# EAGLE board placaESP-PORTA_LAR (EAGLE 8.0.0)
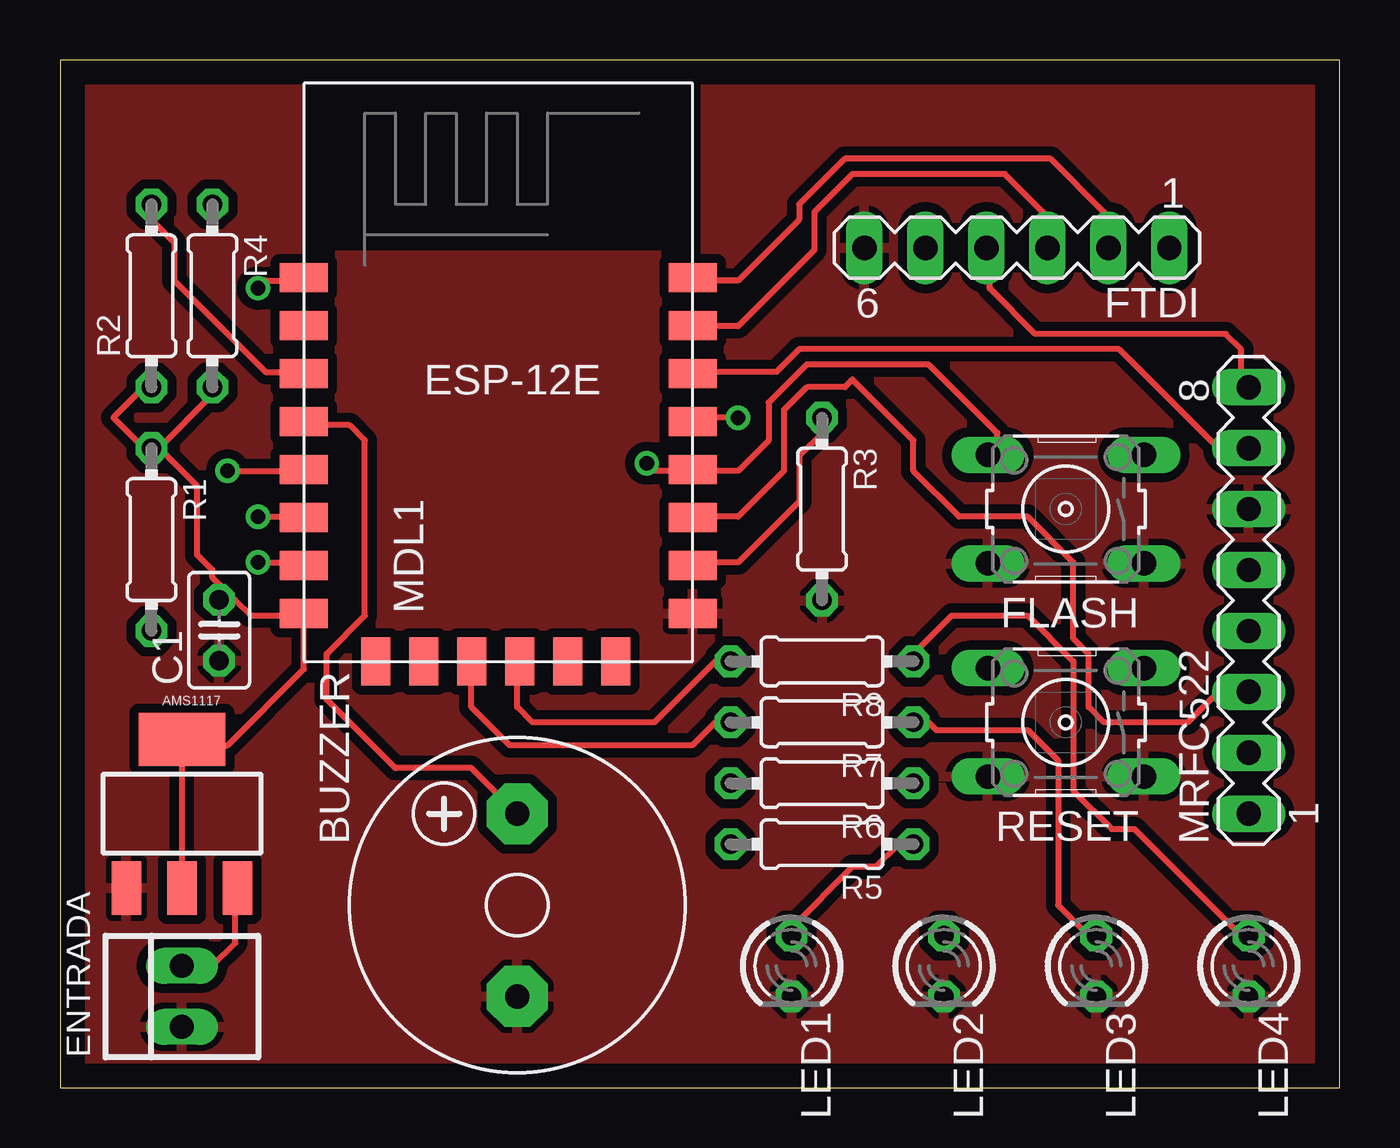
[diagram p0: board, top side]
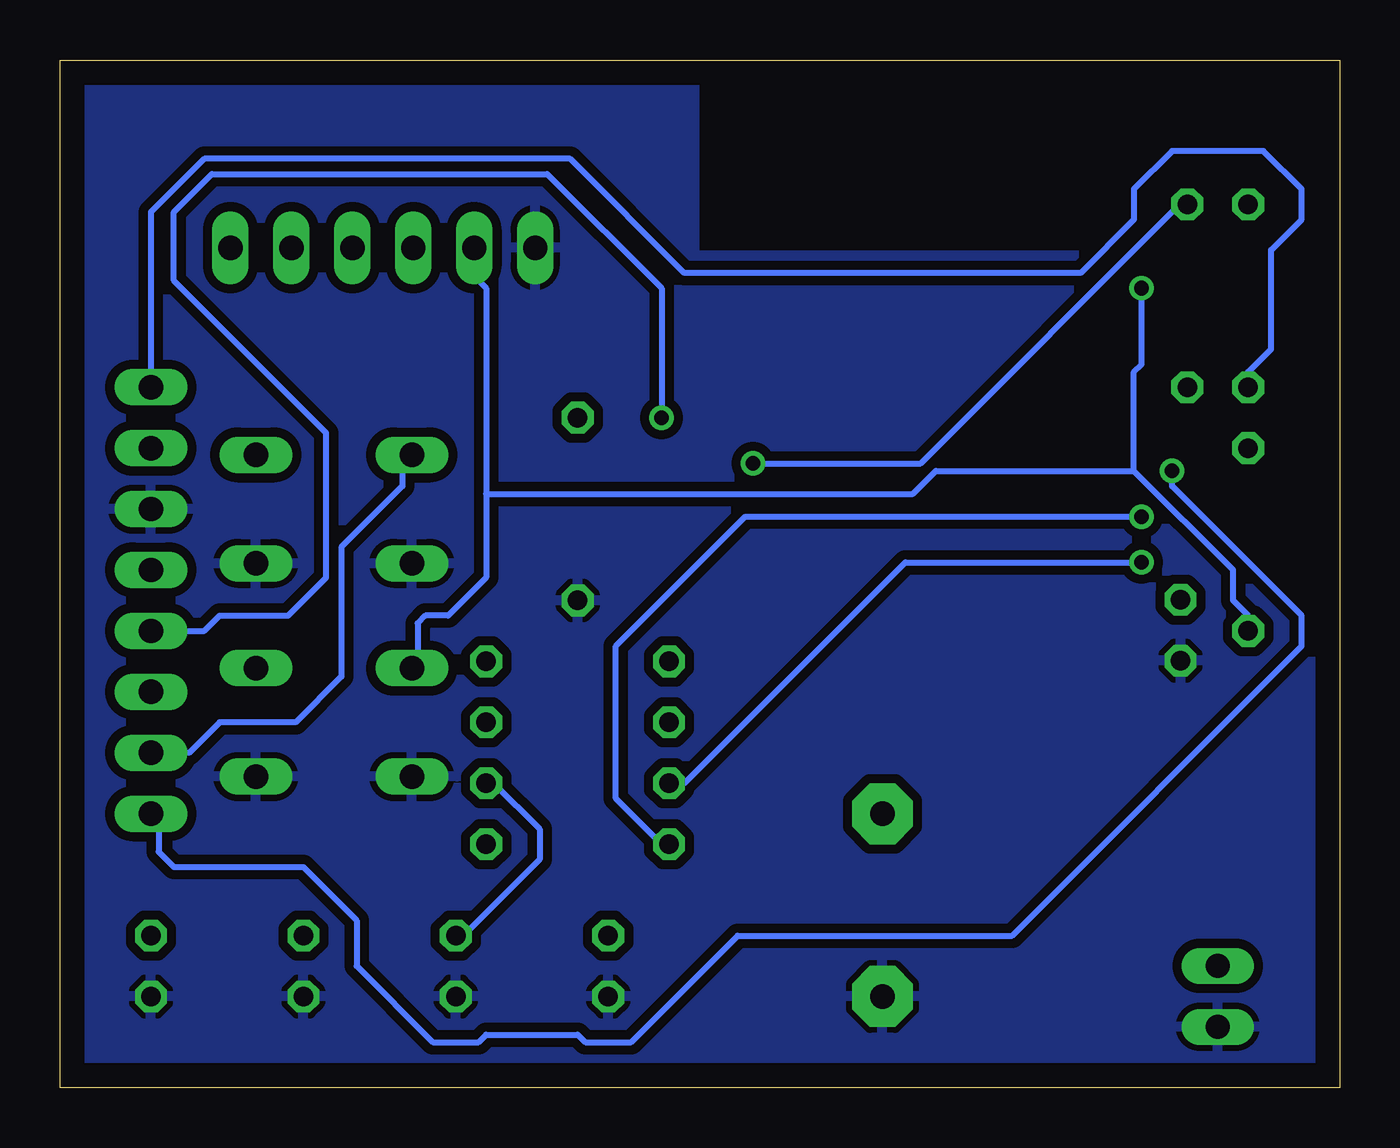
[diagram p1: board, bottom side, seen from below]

Size 53.32 x 42.85 mm. Coordinates in mm from the lower left corner, seen from the top.
Outline: 0,0 53.32,0 53.32,42.85 0,42.85 0,0
Copper layers (1*16): Top 0.035mm / dielectric 1.5mm / Bottom 0.035mm
Design rules "default *": minimum track width 10mil, minimum drill 24mil, track to track 15mil, track to pad 15mil, pad to pad 15mil, via to via 15mil, smd to smd 8mil, copper to edge 40mil, drill to drill 8mil, minimum pad ring 10mil, minimum via ring 8mil, stop-mask expansion 4mil, vias tented up to drill 0mil, thermal gap 10mil

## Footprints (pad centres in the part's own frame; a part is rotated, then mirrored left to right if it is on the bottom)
AMS1117 = smd 1.219 x 2.235: GND -2.311,-3.099; VIN 2.311,-3.099; VOUT 0,-3.099 | smd 3.6 x 2.2: HEATSINK 0,3.099
F/CM12P = drill 1.016 pad 2.54 octagon: + 3.81,0; - -3.81,0
C025-025X050 = drill 0.813 octagon: 1 -1.27,0; 2 1.27,0
22-23-2021 = drill 1 long: 1 -1.27,0; 2 1.27,0
B3F-10XX = drill 1.016 long: 1 -3.251,2.261; 2 3.251,2.261; 3 -3.251,-2.261; 4 3.251,-2.261
MA06-1 = drill 1.016 long: 1 -6.35,0; 2 -3.81,0; 3 -1.27,0; 4 1.27,0; 5 3.81,0; 6 6.35,0
LED3MM = drill 0.813 octagon: A -1.27,0; K 1.27,0
ESP8266-ESP12E = smd 2 x 1.2: 1 -7.62,5.84; 2 -7.62,3.84; 3 -7.62,1.84; 4 -7.62,-0.16; 5 -7.62,-2.16; 6 -7.62,-4.16; 7 -7.62,-6.16; 8 -7.62,-8.16; 9 8.58,-8.16; 10 8.58,-6.16; 11 8.58,-4.16; 12 8.58,-2.16; 13 8.58,-0.16; 14 8.58,1.84; 15 8.58,3.84; 16 8.58,5.84 | smd 1.2 x 2: 17 -4.62,-10.16; 18 -2.62,-10.16; 19 -0.62,-10.16; 20 1.38,-10.16; 21 3.38,-10.16; 22 5.38,-10.16
MA08-1 = drill 1.016 long: 1 -8.89,0; 2 -6.35,0; 3 -3.81,0; 4 -1.27,0; 5 1.27,0; 6 3.81,0; 7 6.35,0; 8 8.89,0
0204/7 = drill 0.813 octagon: 1 -3.81,0; 2 3.81,0

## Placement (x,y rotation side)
AMS1117  [AMS1117]  5.08,11.43 0 top
BUZZER  F/CM12P  [F/CM12P]  19.05,7.62 90 top
C1  100n  [C025-025X050]  6.63,19.08 90 top
ENTRADA  22-23-2021  [22-23-2021]  5.08,3.81 90 top
FLASH  [B3F-10XX]  41.91,24.13 180 top
FTDI  [MA06-1]  39.87,35.02 180 top
LED1  [LED3MM]  30.48,5.08 270 top
LED2  [LED3MM]  36.83,5.08 270 top
LED3  [LED3MM]  43.18,5.08 270 top
LED4  [LED3MM]  49.53,5.08 270 top
MDL1  [ESP8266-ESP12E]  17.78,27.94 0 top
MRFC522  [MA08-1]  49.53,20.32 90 top
R1  10k  [0204/7]  3.81,22.86 270 top
R2  10k  [0204/7]  3.81,33.02 90 top
R3  10k  [0204/7]  31.75,24.13 270 top
R4  10k  [0204/7]  6.35,33.02 270 top
R5  220R  [0204/7]  31.75,10.16 180 top
R6  220R  [0204/7]  31.75,12.7 180 top
R7  220R  [0204/7]  31.75,15.24 180 top
R8  220R  [0204/7]  31.75,17.78 180 top
RESET  [B3F-10XX]  41.91,15.24 180 top

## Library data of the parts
AMS1117 = kaibader
BUZZER = buzzer; OC_FARNELL: unknown; OC_NEWARK: unknown
C1 = rcl
ENTRADA = con-molex; MF: MOLEX; MPN: 22-23-2021; OC_FARNELL: 1462926; OC_NEWARK: 25C3832
FLASH RESET = switch-omron; MPN: B3F-1000; OC_FARNELL: 176432; OC_NEWARK: 36M3542
FTDI MRFC522 = con-lstb; OC_FARNELL: unknown; OC_NEWARK: unknown
LED1-LED4 = led
MDL1 = ESP8266-ESP12E
R1-R8 = resistor

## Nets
BUZZ: BUZZER.+ MDL1.4
CTS: FTDI.5 MDL1.1 R1.2 RESET.4
DTR: FTDI.1
GND: AMS1117.GND BUZZER.- C1.1 ENTRADA.1 FLASH.1 FLASH.2 FTDI.6 LED1.K LED2.K LED3.K LED4.K MDL1.9 MRFC522.6 R3.2 RESET.1 RESET.2
IN+: AMS1117.VIN ENTRADA.2
IRQ: MRFC522.5
LED1: MDL1.6 R5.2
LED2: MDL1.7 R6.2
LED3: MDL1.19 R7.2
LED4: MDL1.20 R8.2
MISO: MDL1.13 MRFC522.4
MOSI: MDL1.11 MRFC522.3
N$1: MDL1.10 R3.1
N$3: MDL1.3 R2.2
N$5: LED1.A R5.1
N$6: LED2.A R6.1
N$7: LED3.A R7.1
N$8: LED4.A R8.1
RST: MDL1.14 MRFC522.7
RXI: FTDI.2 MDL1.16
SCK: FLASH.4 MDL1.12 MRFC522.2 R4.1
SDA: MDL1.5 MRFC522.1
TXO: FTDI.3 MDL1.15
VCC: AMS1117.HEATSINK AMS1117.VOUT C1.2 FTDI.4 MDL1.8 MRFC522.8 R1.1 R2.1 R4.2

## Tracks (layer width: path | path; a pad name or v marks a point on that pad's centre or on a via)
BUZZ
  Top 0.254: BUZZER.+ 17.14,13.34 13.97,13.34 11.11,16.19 11.11,18.1 12.7,19.68 12.7,26.99 12.06,27.62 10.16,27.62 MDL1.4
CTS  (via drill 0.61)
  Top 0.254: v8.26,33.34 8.57,33.66 10.16,33.66 MDL1.1
  Bottom 0.254: v8.26,33.34 8.26,30.16 8.57,29.84 8.57,25.72 | 8.57,25.72 4.45,21.59 4.45,20.32 3.81,19.68 R1.2 | 35.56,24.77 35.56,33.34 35.88,33.66 35.88,34.92 FTDI.5 | 35.56,24.77 35.56,21.27 37.15,19.68 38.1,19.68 38.42,19.37 38.42,17.78 RESET.4 | 8.57,25.72 16.83,25.72 17.78,24.77 35.56,24.77
GND
  pour Bottom: 0,0 53.35,0 53.35,42.79 0,42.79
  pour Top: 0,0 53.3,0 53.3,42.84 0,42.84
IN+
  Top 0.254: ENTRADA.2 6.35,5.08 7.3,6.03 7.3,8.26 AMS1117.VIN
LED1  (via drill 0.61)
  Top 0.254: v8.26,23.81 10.16,23.81 MDL1.6
  Bottom 0.254: v8.26,23.81 24.77,23.81 30.16,18.41 30.16,12.06 28.26,10.16 R5.2
LED2  (via drill 0.61)
  Top 0.254: v8.26,21.91 10.16,21.91 MDL1.7
  Bottom 0.254: v8.26,21.91 18.1,21.91 27.3,12.7 R6.2
LED3
  Top 0.254: R7.2 27.3,15.24 26.35,14.29 18.73,14.29 17.14,15.88 17.14,17.78 MDL1.19
LED4
  Top 0.254: R8.2 27.3,17.78 24.77,15.24 19.68,15.24 19.05,15.88 19.05,17.78 MDL1.20
MISO  (via drill 0.61)
  Top 0.254: v28.26,27.94 26.67,27.94 MDL1.13
  Bottom 0.254: v28.26,27.94 28.26,33.34 33.02,38.1 46.99,38.1 48.58,36.51 48.58,33.66 42.23,27.3 42.23,21.27 43.81,19.68 46.67,19.68 47.31,19.05 MRFC522.4
MOSI
  Top 0.254: MRFC522.3 48.26,16.51 46.99,15.24 43.5,15.24 42.86,15.88 42.86,18.1 42.23,18.73 42.23,21.91 40.32,23.81 37.47,23.81 35.56,25.72 35.56,26.99 33.02,29.53 32.7,29.21 31.11,29.21 30.16,28.26 30.16,25.72 28.26,23.81 26.67,23.81 MDL1.11
N$1
  Top 0.254: R3.1 31.75,27.3 30.8,26.35 30.8,24.45 28.26,21.91 26.67,21.91 MDL1.10
N$3
  Top 0.254: R2.2 3.81,36.2 4.76,35.24 4.76,33.66 8.57,29.84 10.16,29.84 MDL1.3
N$5
  Top 0.254: LED1.A 30.48,6.67 33.02,9.21 33.97,9.21 34.92,10.16 R5.1
N$6
  Bottom 0.254: LED2.A 36.51,6.35 33.34,9.53 33.34,10.79 35.24,12.7 R6.1
N$7
  Top 0.254: LED3.A 42.86,6.35 41.59,7.62 41.59,13.65 40.32,14.92 36.51,14.92 36.2,15.24 R7.1
N$8
  Top 0.254: LED4.A 49.21,6.35 44.77,10.79 43.81,10.79 42.23,12.38 42.23,17.78 40.32,19.68 37.15,19.68 35.56,18.1 R8.1
RST
  Top 0.254: MRFC522.7 48.26,26.67 44.13,30.8 30.8,30.8 29.84,29.84 26.67,29.84 MDL1.14
RXI
  Top 0.254: MDL1.16 26.67,33.66 28.26,33.66 30.8,36.2 30.8,36.83 32.7,38.73 41.27,38.73 43.5,36.51 43.5,35.24 FTDI.2
SCK  (via drill 0.61)
  Top 0.254: FLASH.4 38.73,26.67 39.05,26.99 39.05,27.3 36.2,30.16 31.11,30.16 29.53,28.57 29.53,26.99 28.26,25.72 26.67,25.72 MDL1.12 26.35,25.72 24.77,25.72 v24.45,26.04
  Bottom 0.254: R4.1 6.67,36.83 17.46,26.04 v24.45,26.04 | MRFC522.2 47.94,13.97 46.67,15.24 43.5,15.24 41.59,17.14 41.59,22.54 39.05,25.08 39.05,26.04 38.73,26.35 FLASH.4
SDA  (via drill 0.61)
  Top 0.254: v6.99,25.72 10.16,25.72 MDL1.5
  Bottom 0.254: v6.99,25.72 6.99,25.08 1.59,19.68 1.59,18.41 13.65,6.35 25.08,6.35 29.53,1.91 31.43,1.91 31.75,2.22 35.56,2.22 35.88,1.91 37.78,1.91 40.96,5.08 40.96,6.99 43.18,9.21 48.58,9.21 49.21,9.84 49.21,11.11 MRFC522.1
TXO
  Top 0.254: MDL1.15 26.67,31.75 28.26,31.75 31.43,34.92 31.43,36.51 33.02,38.1 39.37,38.1 40.96,36.51 40.96,35.24 FTDI.3
VCC
  Top 0.254: MRFC522.8 49.21,29.53 49.21,30.8 48.58,31.43 40.64,31.43 38.73,33.34 38.73,34.92 FTDI.4 | 4.13,26.67 6.35,28.89 R4.2 | R2.1 3.49,29.21 2.22,27.94 3.49,26.67 R1.1 4.13,26.67 | 10.16,19.68 7.94,19.68 7.3,20.32 | 7.3,20.32 6.67,20.32 C1.2 | 5.08,14.29 AMS1117.VOUT | 10.16,19.68 10.16,17.46 6.99,14.29 5.08,14.29 | 10.16,19.68 MDL1.8 | 5.08,14.29 AMS1117.HEATSINK | 4.13,26.67 5.71,25.08 5.71,22.23 6.35,21.59 6.35,21.27 7.3,20.32
  Bottom 0.254: MRFC522.8 49.53,36.51 47.31,38.73 32.07,38.73 27.3,33.97 10.79,33.97 8.57,36.2 8.57,37.47 6.99,39.05 3.17,39.05 1.59,37.47 1.59,36.2 2.86,34.92 2.86,30.8 3.81,29.84 R2.1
